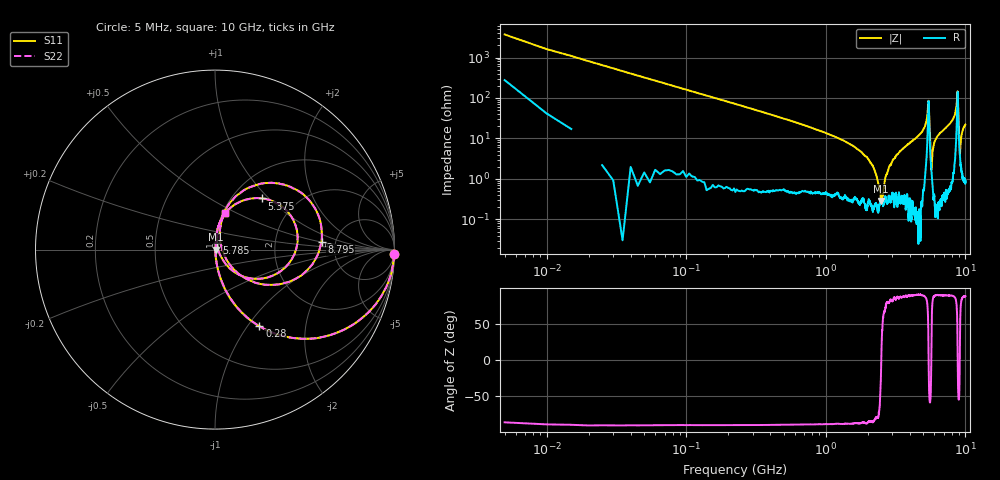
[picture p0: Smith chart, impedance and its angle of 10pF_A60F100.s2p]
! Amotech Co.,Ltd.
! http://www.amotech.co.kr/
! Part Number: A60F100
! These Parameters are Measured in Series Mode Connection
! Operation Temp=25[degC], DC Bias Voltage=0[V]
! Freq. Start=5[MHz] Stop=10[GHz], 2000[Steps]
! Date: Monday, July 20, 2020, 03:34:03
# GHZ S RI R 50.000000
!Freq.(Hz) S11(Real) S11(Imag) S21(Real) S21(Imag) S12(Real) S12(Imag) S22(Real) S22(Imag)
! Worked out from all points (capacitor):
!   2000 points, 5 MHz to 10 GHz, reference 50 ohm
!   read as one part in series: C = 9.9 pF near 55 MHz
!   lowest |Z| = 288 mohm at 2.495 GHz (marker M1)
!   series resonance near 2.496 GHz, so ESL is about 410 pH
!   S11 on the Smith chart (normalised r, x): 5 MHz: 7, -74; 280 MHz: 1.01, -1.14; 5.375 GHz: 1.36, +0.91; 5.785 GHz: 1.02, +0.07; 8.795 GHz: 3.87, +0.51; 10 GHz: 1.02, +0.44
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0.005  0.9973 -0.0268  0.00273 0.0268  0.00273 0.0268  0.9973 -0.0268
0.095  0.739 -0.4346  0.261 0.4346  0.261 0.4346  0.739 -0.4346
0.28  0.2469 -0.4263  0.7531 0.4263  0.7531 0.4263  0.2469 -0.4263
1.675  0.00607 -0.0546  0.9939 0.0546  0.9939 0.0546  0.00607 -0.0546
2.19  0.00232 -0.0194  0.9977 0.0194  0.9977 0.0194  0.00232 -0.0194
2.495  0.00287 -8.07e-05  0.9971 8.07e-05  0.9971 8.07e-05  0.00287 -8.07e-05
2.845  0.00429 0.0198  0.9957 -0.0198  0.9957 -0.0198  0.00429 0.0198
3.34  0.00662 0.044  0.9934 -0.044  0.9934 -0.044  0.00662 0.044
5.005  0.0319 0.1604  0.9681 -0.1604  0.9681 -0.1604  0.0319 0.1604
5.375  0.2629 0.2853  0.7371 -0.2853  0.7371 -0.2853  0.2629 0.2853
5.485  0.3184 -0.1464  0.6816 0.1464  0.6816 0.1464  0.3184 -0.1464
5.69  0.0177 -0.00219  0.9823 0.00219  0.9823 0.00219  0.0177 -0.00219
5.785  0.0106 0.035  0.9894 -0.035  0.9894 -0.035  0.0106 0.035
6.025  0.00949 0.0837  0.9905 -0.0837  0.9905 -0.0837  0.00949 0.0837
6.67  0.0226 0.1385  0.9774 -0.1385  0.9774 -0.1385  0.0226 0.1385
8.335  0.1286 0.3067  0.8714 -0.3067  0.8714 -0.3067  0.1286 0.3067
8.66  0.3741 0.3639  0.6259 -0.3639  0.6259 -0.3639  0.3741 0.3639
8.795  0.5935 0.043  0.4065 -0.043  0.4065 -0.043  0.5935 0.043
8.9  0.2888 -0.1962  0.7112 0.1962  0.7112 0.1962  0.2888 -0.1962
9.135  0.0368 0.0135  0.9632 -0.0135  0.9632 -0.0135  0.0368 0.0135
9.44  0.0306 0.1275  0.9694 -0.1275  0.9694 -0.1275  0.0306 0.1275
10  0.0538 0.2064  0.9462 -0.2064  0.9462 -0.2064  0.0538 0.2064
